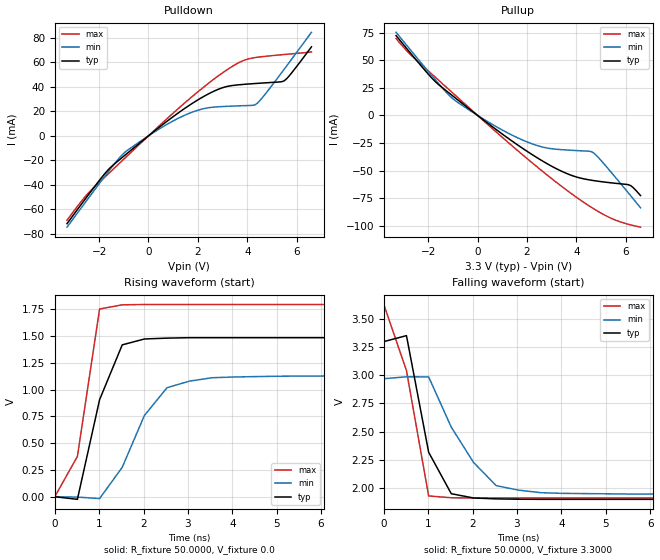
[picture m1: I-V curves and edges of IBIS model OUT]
| SEIKO EPSON CORPORATION
| IBIS file vg7050can2.ibs for VG7050CAN (40MHz to 80MHz)
[IBIS ver] 3.2
[File name] vg7050can2.ibs
[File Rev] 1.0
[Date]  Apr 4 2014
[Source] This file originated at SEIKO EPSON Corporation.
[Notes]  1) Only OUT pin is reported in this file,
   VC pins as NC.
   2) Waveforms coming from the model may differ from
   those of actual ICs.
[Disclaimer]  This information is for modeling purposes only and
   is not guaranteed.
[Copyright] Copyright 2014, SEIKO EPSON Corporation,
   All Rights Reserved.
|   Component VG7050CAN
[Component] VG7050CAN
[Manufacturer] SEIKO EPSON
[Package]
| variable   typ   min   max
R_pkg   0.224   NA   NA
L_pkg   5.50n   NA   NA
C_pkg   1.45p   NA   NA
[Pin]  signal_name   model_name   R_pin   L_pin   C_pin
6   vdd   POWER   NA   NA   NA
5   nc   NC   NA   NA   NA
4   out   OUT   0.224   5.50n   1.45p
3   vss   GND   NA   NA   NA
2   oe   NC   NA   NA   NA
1   vc   NC   NA   NA   NA
| Models and submodels in the file (1): OUT (Output)
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|   Model OUT
[Model]  OUT
Model_type Output
Polarity   Inverting
C_comp   1pF   1pF   1pF
[Temperature Range]   25.0000   85.0000   -40.0000
[Voltage Range]   3.3000V   2.9700V   3.6300V
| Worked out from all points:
|   slope of the pulldown table from 0 to 0.495 V, typ, clamps not added: 62.2 ohm
|   slope of the pullup table from 0 to 0.495 V, typ, clamps not added: 58.3 ohm
|   rising waveform, R_fixture 50.0000, V_fixture 0.0: 20-80 % time 608ps typ, 867ps min, 408ps max; typ from 0 V to 1.49 V
|   falling waveform, R_fixture 50.0000, V_fixture 3.3000: 20-80 % time 530ps typ, 947ps min, 565ps max; typ from 3.3 V to 1.9 V
[Pulldown]
|Voltage   I(typ)   I(min)   I(max)
-3.3V     -71.58mA   -74.44mA   -68.79mA
-2.5V     -49.86mA   -52.62mA   -48.03mA
-1.7V     -29.19mA   -31.14mA   -32.34mA
-900mV    -14.89mA   -12.51mA   -17.1mA
400mV     6.455mA    5.175mA    7.522mA
1.4V      21.43mA    16.17mA    25.65mA
2.2V      31.69mA    21.98mA    39.19mA
3.1V      39.85mA    23.98mA    52.77mA
3.8V      41.88mA    24.54mA    61.03mA
4.4V      42.77mA    26.45mA    64.05mA
5.5V      44.91mA    54.46mA    66.33mA
6.6V      72.57mA    84.4mA     68.51mA
[Pullup]
|Voltage   I(typ)   I(min)   I(max)
-3.3V     72.31mA    75.27mA    69.64mA
-2.7V     56.02mA    58.89mA    54.76mA
-1.8V     32.62mA    34.64mA    36.38mA
-1V       17.55mA    15.07mA    20.18mA
700mV     -11.93mA   -9.485mA   -13.95mA
2.1V      -33.94mA   -24.89mA   -40.9mA
2.8V      -43.55mA   -29.52mA   -53.72mA
3.6V      -52.57mA   -31.36mA   -67.6mA
4.7V      -59.08mA   -34.02mA   -84.59mA
5.4V      -61.1mA    -51.25mA   -93.12mA
6.1V      -62.79mA   -70.09mA   -98.66mA
6.6V      -72.68mA   -83.71mA   -101.3mA
[Ramp]
| variable   typ   min   max
dV/dt_r  0.8910/0.6026n   0.6762/0.8597n   1.0770/0.4080n
dV/dt_f  0.8418/0.5267n   0.6156/0.9381n   1.0326/0.5610n
R_load = 50.0000
[Rising Waveform]
R_fixture= 50.0000
V_fixture= 0.0
V_fixture_min= 0.0
V_fixture_max= 0.0
|time   V(typ)   V(min)   V(max)
0s        0V         0V         0V
510ps     -24.35mV   -3.402mV   376.4mV
1.01ns    906.3mV    -17.31mV   1.753V
1.52ns    1.418V     274.6mV    1.792V
2.02ns    1.473V     758.8mV    1.795V
2.53ns    1.481V     1.018V     1.795V
3.03ns    1.485V     1.079V     1.795V
3.54ns    1.485V     1.111V     1.795V
5.56ns    1.485V     1.127V     1.795V
50ns      1.485V     1.127V     1.795V
[Falling Waveform]
R_fixture= 50.0000
V_fixture= 3.3000
V_fixture_min= 2.9700
V_fixture_max= 3.6300
|time   V(typ)   V(min)   V(max)
0s        3.3V       2.97V      3.63V
510ps     3.353V     2.987V     3.042V
1.01ns    2.316V     2.986V     1.927V
1.52ns    1.947V     2.539V     1.911V
2.02ns    1.909V     2.226V     1.909V
2.53ns    1.901V     2.019V     1.909V
3.03ns    1.898V     1.979V     1.909V
3.54ns    1.897V     1.956V     1.909V
5.56ns    1.897V     1.944V     1.909V
50ns      1.897V     1.944V     1.909V
